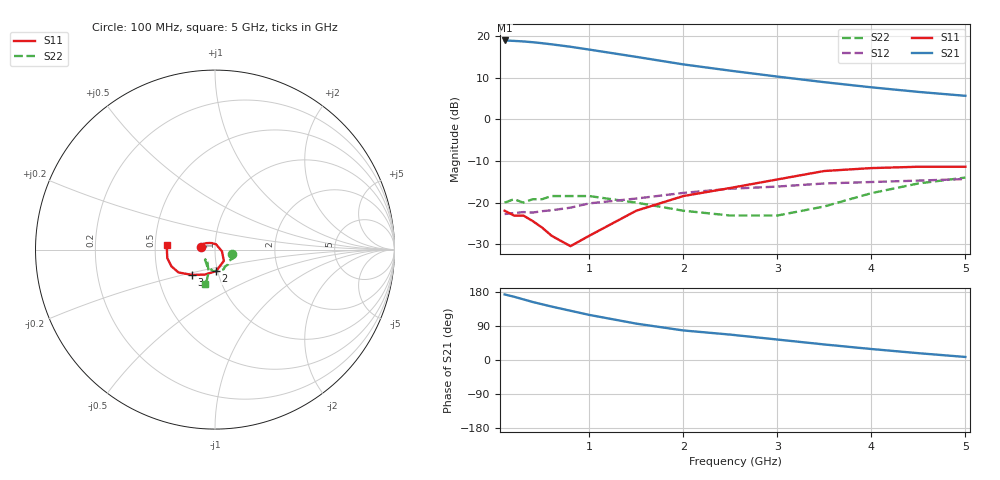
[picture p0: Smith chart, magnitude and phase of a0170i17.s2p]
!  MSA-0170 S AND NOISE PARAMETERS
!  Id=17mA  LAST UPDATED 05-01-90
# ghz s ma r 50
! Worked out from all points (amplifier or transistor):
!   16 points, 100 MHz to 5 GHz, reference 50 ohm
!   highest |S21| = 19.0 dB at 100 MHz (marker M1)
!   |S21| within 3 dB of that: start of sweep to 1.231 GHz
!   unconditionally stable (mu >= 1): start of sweep to end of sweep
!   at 300 MHz: K = 1.07, MAG = 18.9 dB, |S12| = -22.3 dB
!   at 1.5 GHz: K = 1.09, MAG = 15.2 dB, |S12| = -19.0 dB
!   at 5 GHz: K = 1.36, MAG = 6.4 dB, |S12| = -14.3 dB
!   lowest NFmin = 5.20 dB at 100 MHz
!   S11 on the Smith chart (normalised r, x): 100 MHz: 0.85, +0.02; 2 GHz: 0.98, -0.24; 3 GHz: 0.75, -0.22; 5 GHz: 0.58, +0.03
0.1  0.08 171.0  8.88 173.0  0.073 2.0  0.1 -13.0
0.2  0.07 161.0  8.77 167.0  0.075 6.0  0.11 -27.0
0.3  0.07 152.0  8.64 160.0  0.077 8.0  0.1 -39.0
0.4  0.06 143.0  8.45 153.0  0.076 11.0  0.11 -49.0
0.5  0.05 133.0  8.23 147.0  0.079 13.0  0.11 -59.0
0.6  0.04 115.0  7.98 141.0  0.081 17.0  0.12 -67.0
0.8  0.03 79.0  7.46 130.0  0.087 20.0  0.12 -83.0
1  0.04 -14.0  6.9 119.0  0.098 23.0  0.12 -96.0
1.5  0.08 -52.0  5.64 96.0  0.112 26.0  0.1 -116.0
2  0.12 -87.0  4.58 78.0  0.131 24.0  0.08 -134.0
2.5  0.15 -112.0  3.85 67.0  0.147 25.0  0.07 -135.0
3  0.19 -132.0  3.27 54.0  0.156 22.0  0.07 -129.0
3.5  0.24 -148.0  2.8 41.0  0.17 18.0  0.09 -117.0
4  0.26 -159.0  2.43 29.0  0.177 13.0  0.13 -106.0
4.5  0.27 -170.0  2.14 18.0  0.184 8.0  0.17 -105.0
5  0.27 175.0  1.92 8.0  0.192 5.0  0.2 -106.0
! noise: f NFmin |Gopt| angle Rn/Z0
0.1  5.2  0.23  2  1.12
0.5  5.3  0.23  9  1.11
1  5.5  0.22  18  1.1
2  5.8  0.2  35  1.05
